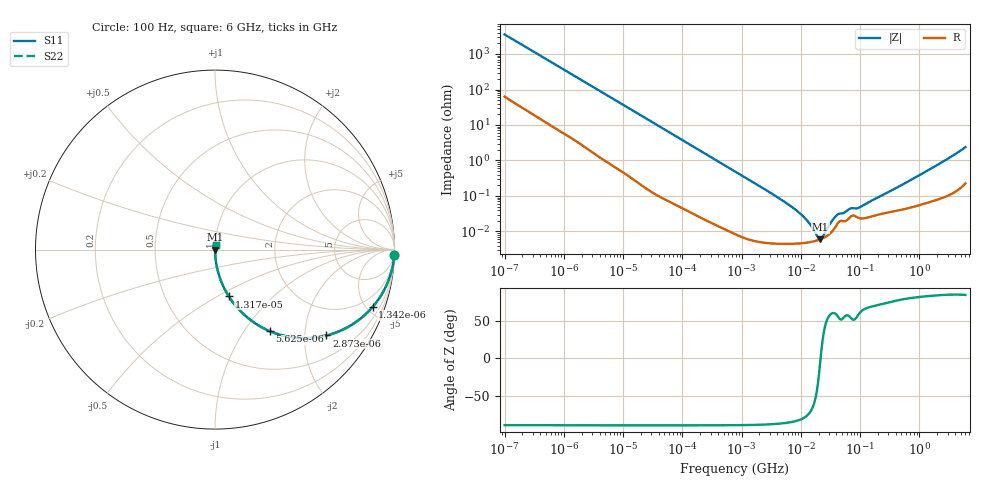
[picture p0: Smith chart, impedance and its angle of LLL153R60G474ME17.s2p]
!Murata Part Number: LLL153R60G474ME17
!These Parameters are Measured in Series Mode Connection
!Data Generated on Mar 13, 2026
!  o--ll--o
!Port1  Port2
!  o------o
!Operation Temp=25[degC], DC Bias Voltage=0[V]
!Freq. Start=100[Hz] Stop=6[GHz] 401[Steps]
# Hz S RI R 50
!Freq.(Hz) S11(Real) S11(Imag) S21(Real) S21(Imag) S12(Real) S12(Imag) S22(Real) S22(Imag)
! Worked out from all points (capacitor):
!   401 points, 100 Hz to 6 GHz, reference 50 ohm
!   read as one part in series: C = 445 nF near 109 Hz
!   lowest |Z| = 6 mohm at 21.28 MHz (marker M1)
!   series resonance near 21.57 MHz, so ESL is about 120 pH
!   S11 on the Smith chart (normalised r, x): 100 Hz: 2, -71; 1.342 kHz: 1.09, -5.45; 2.873 kHz: 1.04, -2.57; 5.625 kHz: 1.02, -1.32; 13.17 kHz: 1.01, -0.57; 6 GHz: 1.00, +0.05
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100  0.9987 -0.028  0.00128 0.028  0.00128 0.028  0.9987 -0.028
419  0.9849 -0.1139  0.0151 0.1139  0.0151 0.1139  0.9849 -0.1139
1342  0.8776 -0.3201  0.1224 0.3201  0.1224 0.3201  0.8776 -0.3201
2008  0.7666 -0.4156  0.2334 0.4156  0.2334 0.4156  0.7666 -0.4156
2873  0.6205 -0.4783  0.3795 0.4783  0.3795 0.4783  0.6205 -0.4783
5625  0.3051 -0.454  0.6949 0.454  0.6949 0.454  0.3051 -0.454
13169  0.077 -0.2607  0.923 0.2607  0.923 0.2607  0.077 -0.2607
40335  0.00955 -0.0922  0.9905 0.0922  0.9905 0.0922  0.00955 -0.0922
774597  0.000108 -0.00495  0.9999 0.00495  0.9999 0.00495  0.000108 -0.00495
6948629  4.5e-05 -0.000498  1 0.000498  1 0.000498  4.5e-05 -0.000498
1.137099e7  4.73e-05 -0.000246  1 0.000246  1 0.000246  4.73e-05 -0.000246
1.555665e7  5.14e-05 -0.00012  0.9999 0.00012  0.9999 0.00012  5.14e-05 -0.00012
1.779312e7  5.42e-05 -7e-05  0.9999 7e-05  0.9999 7e-05  5.42e-05 -7e-05
2.128304e7  5.98e-05 -4.8e-06  0.9999 4.8e-06  0.9999 4.8e-06  5.98e-05 -4.8e-06
2.662322e7  7.18e-05 7.81e-05  0.9999 -7.81e-05  0.9999 -7.81e-05  7.18e-05 7.81e-05
3.64232e7  0.000117 0.000205  0.9999 -0.000205  0.9999 -0.000205  0.000117 0.000205
4.35672e7  0.000182 0.000254  0.9998 -0.000254  0.9998 -0.000254  0.000182 0.000254
6.817316e7  0.000254 0.00036  0.9997 -0.00036  0.9997 -0.00036  0.000254 0.00036
9.753859e7  0.000237 0.000411  0.9998 -0.000411  0.9998 -0.000411  0.000237 0.000411
3.124326e8  0.00035 0.00128  0.9996 -0.00128  0.9996 -0.00128  0.00035 0.00128
1.791126e9  0.000779 0.00663  0.9992 -0.00663  0.9992 -0.00663  0.000779 0.00663
6e9  0.00282 0.0236  0.9972 -0.0236  0.9972 -0.0236  0.00282 0.0236
